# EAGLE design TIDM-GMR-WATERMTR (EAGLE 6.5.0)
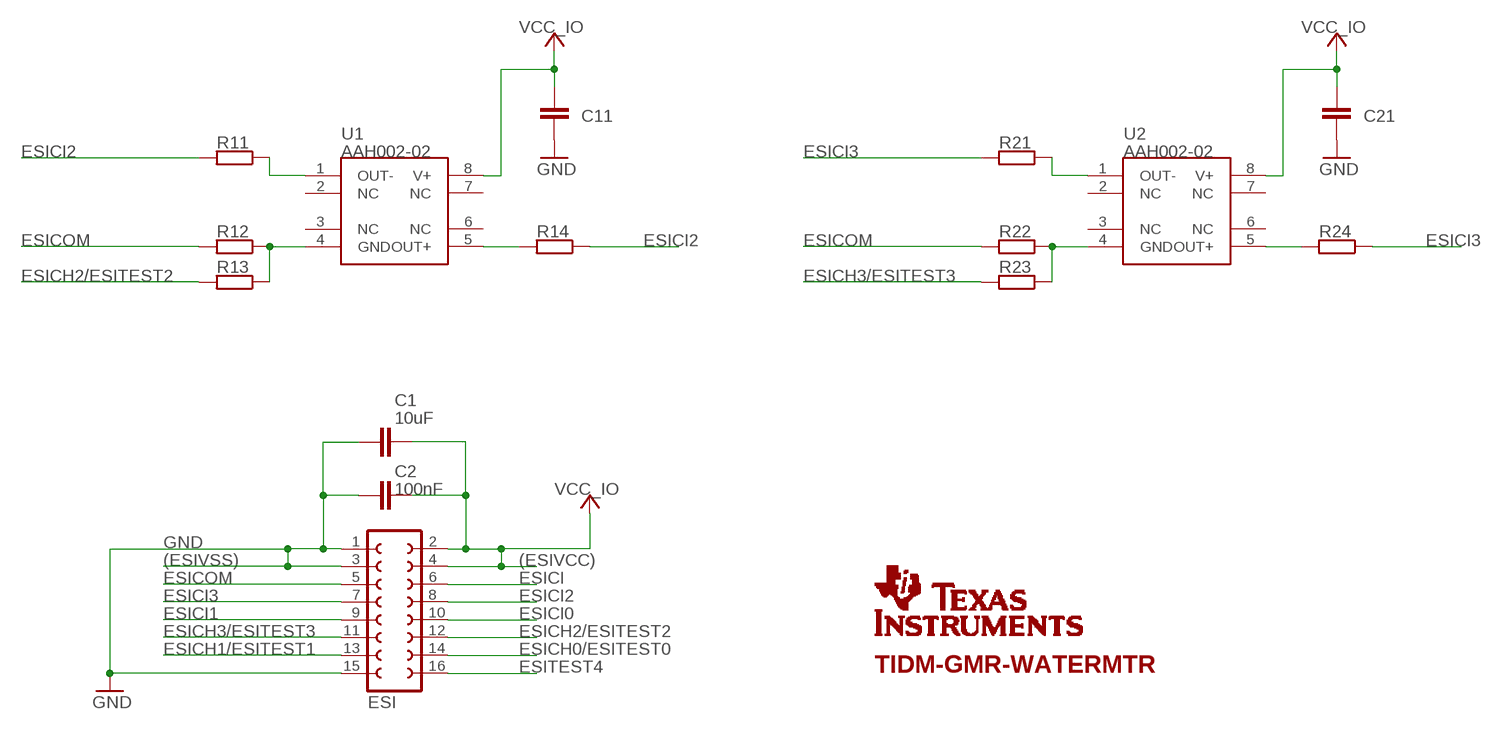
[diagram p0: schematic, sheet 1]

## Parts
C1  10uF  C-EUC0805  [C0805]
C2  100nF  C-EUC0402  [C0402]
C11  C-EUC0402  [C0402]
C21  C-EUC0402  [C0402]
ESI  FE08-2  [FE08-2]
R11  R-EU_R0402  [R0402]
R12  R-EU_R0402  [R0402]
R13  R-EU_R0402  [R0402]
R14  R-EU_R0402  [R0402]
R21  R-EU_R0402  [R0402]
R22  R-EU_R0402  [R0402]
R23  R-EU_R0402  [R0402]
R24  R-EU_R0402  [R0402]
U1  AAH002-02  [SO-08]
U2  AAH002-02  [SO-08]
U$1  TI-LOGO-SMALL  [TI-LOGO-4]

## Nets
ESICH0/ESITEST0: ESI.14
ESICH1/ESITEST1: ESI.13
ESICH2/ESITEST2: ESI.12 R13.2
ESICH3/ESITEST3: ESI.11 R23.2
ESICI: ESI.6
ESICI0: ESI.10
ESICI1: ESI.9
ESICI2: ESI.8 R11.2 R14.1
ESICI3: ESI.7 R21.2 R24.1
ESICOM: ESI.5 R12.2 R22.2
ESITEST4: ESI.16
GND: C1.2 C2.2 C11.2 C21.2 ESI.1 ESI.3 ESI.15
N$3: R11.1 U1.1(OUT-)
N$4: R14.2 U1.5(OUT+)
N$13: R22.1 R23.1 U2.4(GND)
N$17: R12.1 R13.1 U1.4(GND)
N$18: R21.1 U2.1(OUT-)
N$19: R24.2 U2.5(OUT+)
VCC_IO: C1.1 C2.1 C11.1 C21.1 ESI.2 ESI.4 U1.8(V+) U2.8(V+)
Unconnected: U1.2(NC) U1.3(NC) U1.6(NC) U1.7(NC) U2.2(NC) U2.3(NC) U2.6(NC) U2.7(NC)

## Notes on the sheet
- (ESIVSS) | (ESIVCC)
- TIDM-GMR-WATERMTR

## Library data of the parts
C1 C2 C11 C21 = rcl:C-EU: CAPACITOR, European symbol
ESI = con-lsta:FE08-2: FEMALE HEADER; OC_FARNELL: unknown; OC_NEWARK: unknown
R11-R14 R21-R24 = rcl:R-EU_: RESISTOR, European symbol
U1 U2 = GMR Sensor:AAH002-02
U$1 = texas-logo:TI-LOGO: Full TI logo

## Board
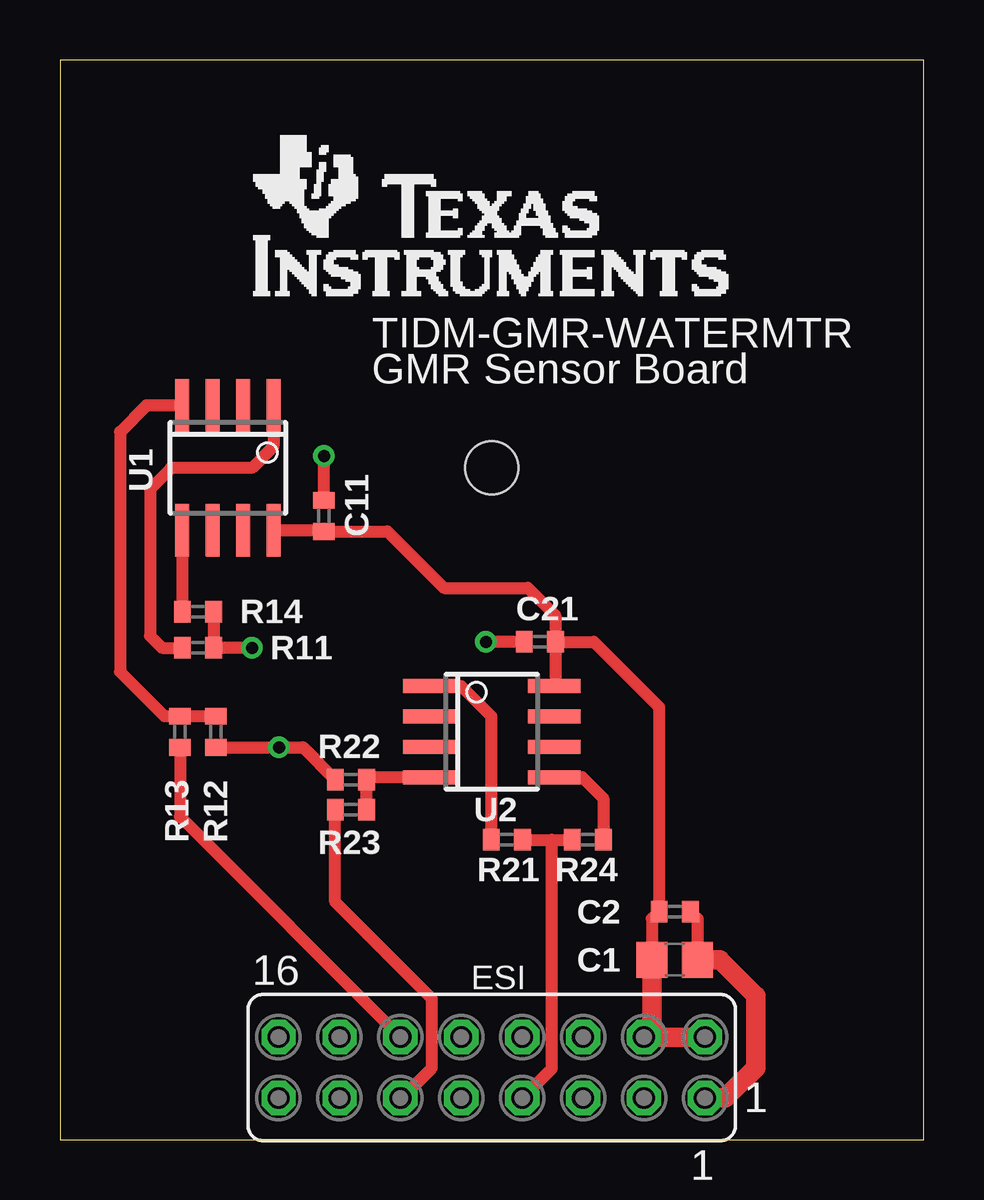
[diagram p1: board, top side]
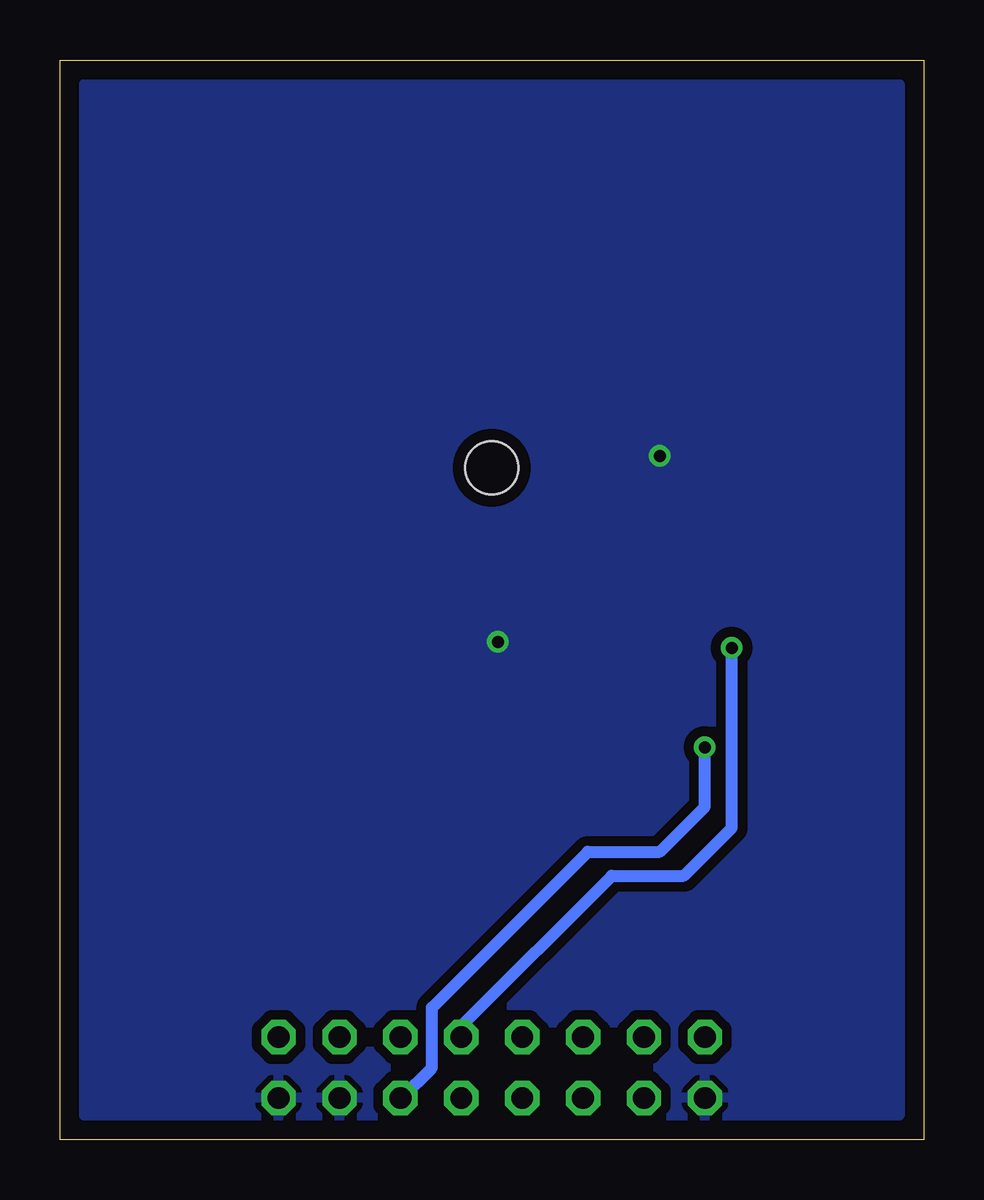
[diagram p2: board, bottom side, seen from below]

Size 36 x 45 mm. Coordinates in mm from the lower left corner, seen from the top.
Outline: 36,0 36,45 0,45 0,0 36,0
Copper layers (1*16): Top 0.035mm / dielectric 1.5mm / Bottom 0.035mm
Design rules "default": minimum track width 10mil, minimum drill 0.3mm, track to track 8mil, track to pad 8mil, pad to pad 8mil, via to via 8mil, smd to smd 8mil, copper to edge 20mil, drill to drill 8mil, minimum pad ring 10mil, minimum via ring 8mil, stop-mask expansion 4mil, vias tented up to drill 100mil, thermal gap 10mil
Holes 2.2 mm at 18,28

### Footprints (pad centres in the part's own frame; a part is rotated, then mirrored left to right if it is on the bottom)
C0805 = smd 1.3 x 1.5: 1 -0.95,0; 2 0.95,0
C0402 = smd 0.7 x 0.9: 1 -0.65,0; 2 0.65,0
FE08-2 = drill 0.914 octagon: 1 -8.89,1.27; 2 -8.89,-1.27; 3 -6.35,1.27; 4 -6.35,-1.27; 5 -3.81,1.27; 6 -3.81,-1.27; 7 -1.27,1.27; 8 -1.27,-1.27; 9 1.27,1.27; 10 1.27,-1.27; 11 3.81,1.27; 12 3.81,-1.27; 13 6.35,1.27; 14 6.35,-1.27; 15 8.89,1.27; 16 8.89,-1.27
R0402 = smd 0.7 x 0.9: 1 -0.65,0; 2 0.65,0
SO-08 = smd 0.6 x 2.2: 1 -1.905,-2.6; 2 -0.635,-2.6; 3 0.635,-2.6; 4 1.905,-2.6; 5 1.905,2.6; 6 0.635,2.6; 7 -0.635,2.6; 8 -1.905,2.6

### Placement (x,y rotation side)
C1  25.62,7.5 0 top
C2  25.62,9.5 0 top
C11  11,26 90 top
C21  20,20.75 180 top
ESI  18,3 180 top
R11  5.75,20.5 0 top
R12  6.5,17 270 top
R13  5,17 270 top
R14  5.75,22 180 top
R21  18.62,12.5 0 top
R22  12.12,15 180 top
R23  12.12,13.75 180 top
R24  22,12.5 0 top
U1  7,28 180 top
U2  18,17 270 top
U$1  8,35 0 top

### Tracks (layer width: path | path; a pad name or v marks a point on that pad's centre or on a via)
ESICH2/ESITEST2
  Top 0.508: R13.2 5,13.46 ESI.12
ESICH3/ESITEST3
  Top 0.508: ESI.11 14.23,1.73 15.5,3 15.5,5.88 11.47,9.9 R23.2
ESICI2  (via drill 0.5)
  Top 0.508: R14.1 R11.2 v8,20.5
  Bottom 0.508: ESI.8 19.27,4.73 13,11 10,11 8,13 v8,20.5
ESICI3
  Top 0.508: R21.2 20.5,12.5 | 20.5,12.5 R24.1 | ESI.7 20.5,2.96 20.5,12.5
ESICOM  (via drill 0.5)
  Top 0.508: R12.2 v9.12,16.35 10.12,16.35 R22.2
  Bottom 0.508: ESI.5 21.77,1.73 20.5,3 20.5,5.5 14,12 11,12 9.12,13.88 v9.12,16.35
GND  (via drill 0.5)
  Top 0.508: C11.2 v11,28.5 | C21.2 v17.75,20.75 | C2.2 26.57,9.2 C1.2
  Top 0.813: C1.2 27.5,7.5 29,6 29,3 27.73,1.73 ESI.1
  pour Bottom (isolate 0.406, rank 2): 1,1 35,1 35,44 1,44
N$3
  Top 0.508: U1.1 8.9,28.91 8,28 4.62,28 3.75,27.12 3.75,21 4.25,20.5 R11.1
N$4
  Top 0.508: U1.5 R14.2
N$13
  Top 0.508: R23.1 R22.1 12.78,15.1 U2.4
N$17
  Top 0.508: U1.4 3.6,30.6 2.5,29.5 2.5,19.5 4.35,17.65 R13.1 R12.1
N$18
  Top 0.508: U2.1 16.72,18.91 17.98,17.65 R21.1
N$19
  Top 0.508: U2.5 21.78,15.1 22.65,14.22 R24.2
VCC_IO
  Top 0.508: U1.8 11,25.4 C11.1 13.65,25.35 16,23 19.5,23 20.65,21.85 C21.1 | C21.1 22.25,20.75 24.98,18.02 C2.1 24.68,9.2 C1.1 | C21.1 20.65,18.91 U2.8
  Top 0.813: ESI.2 ESI.4 24.68,4.27 C1.1

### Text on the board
tPlace: TIDM-GMR-WATERMTR | GMR Sensor Board | 1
